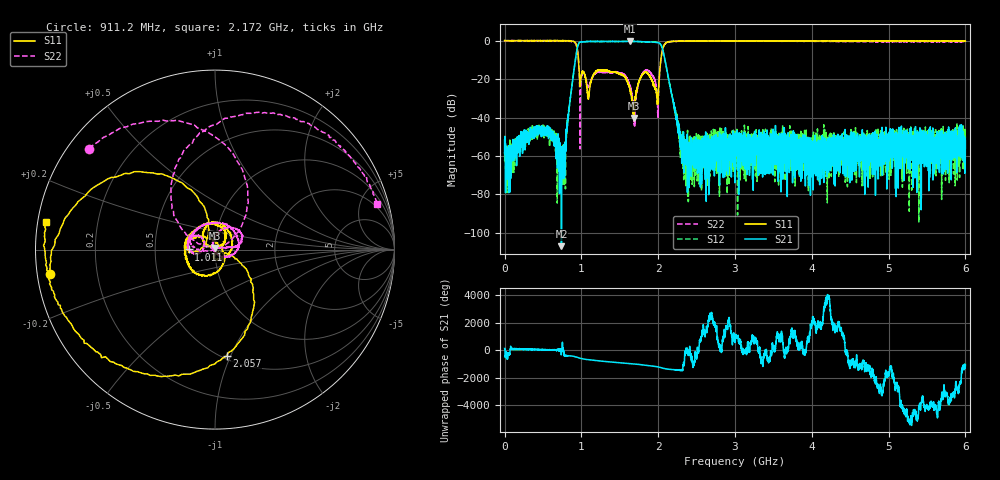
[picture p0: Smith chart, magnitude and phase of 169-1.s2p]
#  HZ  S  MA  R  50.00
! Rohde & Schwarz Vector Network Analyzer
! Rohde-Schwarz,ZNL6-2Port,1323001206101378,1.50.1.34-21.10.1.104
! Created: UTC 4/7/2024, 3:34:05 AM
! freq[Hz]  mag:S11  ang:S11  mag:S21  ang:S21  mag:S12  ang:S12  mag:S22  ang:S22
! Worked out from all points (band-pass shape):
!   6000 points, 5 kHz to 6 GHz, reference 50 ohm
!   highest |S21| = -0.31 dB at 1.637 GHz (marker M1); lowest = -107.0 dB at 740.1 MHz (marker M2)
!   |S21| within 3 dB of the highest: 949.5 MHz to 2.049 GHz (1.1 GHz wide, 73.3 % of centre)
!   lowest |S11| = -40.2 dB at 1.68 GHz (marker M3), VSWR 1.02, Z = 50.1 + j0.97 ohm
!   |S11| at or under -10 dB: 962.2 MHz to 2.034 GHz (1.072 GHz wide, 71.6 % of centre)
!   |S22| runs from -56.3 to 0.1 dB; largest |S21 - S12| = 0.024
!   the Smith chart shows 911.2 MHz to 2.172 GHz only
!   S11 on the Smith chart (normalised r, x): 911.2 MHz: 0.04, -0.07; 1.011 GHz: 0.74, +0.00; 2.057 GHz: 0.53, -0.97; 2.172 GHz: 0.02, +0.08
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5000  1.003 -0.1  0.002641 124.6  0.001277 -67.9  0.9961 -0.9
4.740836e8  0.9974 -42.6  0.004317 39.2  0.004442 37.0  0.9904 -70.4
7.401277e8  1.001 -88.2  4.486e-06 114.9  0.0007833 -146.3  0.9812 -129.8
9.111561e8  0.9298 -171.5  0.2243 -105.1  0.2232 -105.8  0.8981 141.3
9.621646e8  0.3168 108.8  0.8323 165.6  0.8297 165.4  0.2994 53.3
1.000171e9  0.1304 -174.5  0.9257 104.1  0.9271 103.4  0.113 177.8
1.011173e9  0.1467 179.6  0.9258 91.2  0.9257 90.3  0.1416 167.3
1.119191e9  0.07723 -48.4  0.9599 -1.2  0.9595 -1.4  0.08655 -167.4
1.275216e9  0.1625 -166.6  0.9499 -91.3  0.9554 -91.7  0.1496 143.6
1.455246e9  0.1465 103.1  0.9563 -178.4  0.9514 -178.0  0.1527 60.2
1.637277e9  0.04942 32.4  0.9653 95.7  0.9585 96.0  0.06656 -34.2
1.680284e9  0.009757 82.6  0.9608 73.9  0.958 74.0  0.01443 -104.2
1.84131e9  0.1543 88.0  0.9293 -16.3  0.9292 -16.2  0.1714 35.9
1.934326e9  0.07812 -23.4  0.9185 -82.5  0.9151 -82.5  0.1188 8.2
2.000337e9  0.03686 -23.3  0.8865 -146.6  0.8869 -146.2  0.02368 147.8
2.057346e9  0.5964 -83.8  0.6036 128.9  0.5841 129.5  0.5835 107.0
2.172365e9  0.9553 170.7  0.04329 29.0  0.043 29.9  0.9382 15.7
2.362397e9  0.9796 120.0  0.001198 20.5  0.0001852 31.1  0.978 -38.1
3.000503e9  0.9859 71.0  0.003558 -97.8  0.002567 -156.0  0.9916 -120.6
4.000668e9  0.9869 51.0  0.002212 -134.0  0.002286 -84.1  0.96 167.5
5.000834e9  0.9769 49.6  0.001302 10.4  0.001787 -61.4  0.9518 116.8
6e9  0.9794 50.0  0.002509 30.7  0.002705 57.4  0.9421 70.6
